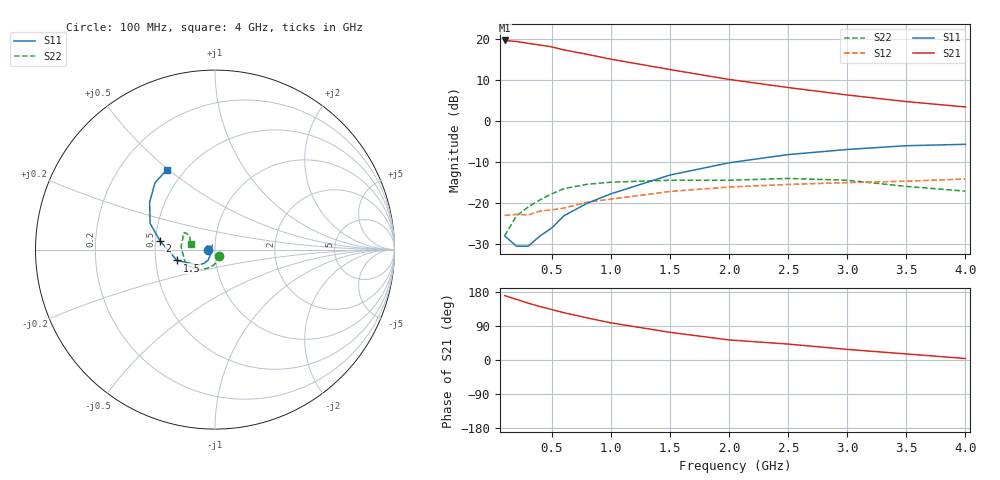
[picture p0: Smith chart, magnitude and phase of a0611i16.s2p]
!  MSA-0611 S AND NOISE PARAMETERS
!  Id=16mA  LAST UPDATED 07-22-92
# ghz s ma r 50
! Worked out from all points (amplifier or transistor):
!   14 points, 100 MHz to 4 GHz, reference 50 ohm
!   highest |S21| = 19.6 dB at 100 MHz (marker M1)
!   |S21| within 3 dB of that: start of sweep to 731.3 MHz
!   unconditionally stable (mu >= 1): start of sweep to end of sweep
!   at 300 MHz: K = 1.10, MAG = 19.0 dB, |S12| = -22.9 dB
!   at 1 GHz: K = 1.06, MAG = 15.5 dB, |S12| = -19.0 dB
!   at 4 GHz: K = 1.37, MAG = 5.1 dB, |S12| = -14.1 dB
!   lowest NFmin = 2.90 dB at 100 MHz
!   S11 on the Smith chart (normalised r, x): 100 MHz: 0.92, -0.01; 1.5 GHz: 0.65, -0.08; 2 GHz: 0.53, +0.06; 4 GHz: 0.40, +0.49
0.1  0.04 -176.0  9.53 170.0  0.071 6.0  0.04 -57.0
0.2  0.03 -163.0  9.25 160.0  0.073 10.0  0.07 -82.0
0.3  0.03 -149.0  8.79 150.0  0.072 14.0  0.09 -97.0
0.4  0.04 -132.0  8.38 141.0  0.08 17.0  0.11 -111.0
0.5  0.05 -127.0  7.96 133.0  0.083 21.0  0.13 -122.0
0.6  0.07 -123.0  7.33 125.0  0.087 23.0  0.15 -131.0
0.8  0.1 -129.0  6.46 111.0  0.103 25.0  0.17 -147.0
1  0.13 -139.0  5.64 98.0  0.112 28.0  0.18 -160.0
1.5  0.22 -164.0  4.22 73.0  0.139 25.0  0.19 175.0
2  0.31 171.0  3.2 53.0  0.157 21.0  0.19 160.0
2.5  0.39 158.0  2.55 42.0  0.169 22.0  0.2 153.0
3  0.45 144.0  2.07 28.0  0.178 18.0  0.19 150.0
3.5  0.5 132.0  1.72 16.0  0.185 15.0  0.16 152.0
4  0.52 121.0  1.48 4.0  0.197 11.0  0.14 166.0
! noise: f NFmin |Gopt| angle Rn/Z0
0.1  2.9  0.12  6  0.41
0.5  3  0.11  28  0.4
1  3.2  0.1  60  0.38
2  3.6  0.11  133  0.34
